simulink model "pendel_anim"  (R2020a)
settings: Solver=ode45  StartTime=0.0  StopTime=30  MaxStep=0.01  RelTol=1e-5  EnableMultiTasking=on

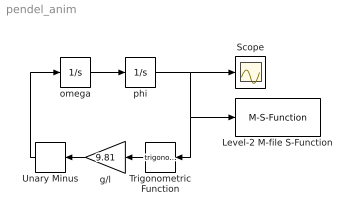
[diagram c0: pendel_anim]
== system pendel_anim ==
  Level-2 M-file S-Function : M-S-Function  FunctionName=sfun_pendelanim
  Scope : Scope
  Trigonometric Function : Trigonometry
  Unary Minus : UnaryMinus
  g/l : Gain  Gain=9.81
  omega : Integrator
  phi : Integrator  InitialCondition=pi*0.999
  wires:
  omega/1 -> phi/1
  phi/1 -> Scope/1, Trigonometric Function/1, Level-2 M-file S-Function/1
  g/l/1 -> Unary Minus/1
  Trigonometric Function/1 -> g/l/1
  Unary Minus/1 -> omega/1
